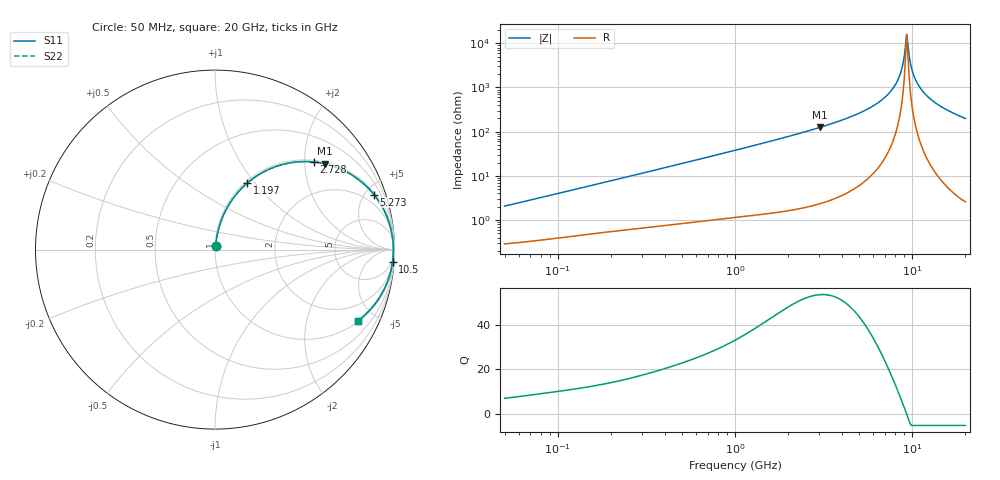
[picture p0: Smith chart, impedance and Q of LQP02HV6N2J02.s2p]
!Murata Part Number: LQP02HV6N2J02
!These Parameters are Measured in Series Mode Connection
!  o--[Z]--o
!Port1  Port2
!  o-------o
!Freq. Start=50[MHz] Stop=20[GHz], 401[Steps]
# Hz S RI R 50
!Freq.(Hz) S11(Real) S11(Imag) S21(Real) S21(Imag) S12(Real) S12(Imag) S22(Real) S22(Imag)
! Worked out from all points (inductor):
!   401 points, 50 MHz to 20 GHz, reference 50 ohm
!   read as one part in series: L = 6.45 nH near 51.52 MHz
!   highest Q = 53.3 at 3.03 GHz (marker M1), where L = 6.6 nH
!   self-resonance near 9.317 GHz
!   S11 on the Smith chart (normalised r, x): 50 MHz: 1.01, +0.04; 1.197 GHz: 1.02, +0.91; 2.728 GHz: 1.04, +2.22; 5.273 GHz: 1.14, +5.74; 10.5 GHz: 4, -29; 20 GHz: 1.05, -3.97
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5e7  0.0033 0.0204  0.9967 -0.0204  0.9967 -0.0204  0.0033 0.0204
1.364002e8  0.0074 0.0531  0.9926 -0.0531  0.9926 -0.0531  0.0074 0.0531
3.721004e8  0.0266 0.1374  0.9734 -0.1374  0.9734 -0.1374  0.0266 0.1374
1e9  0.1329 0.3247  0.8671 -0.3247  0.8671 -0.3247  0.1329 0.3247
1.196911e9  0.178 0.3691  0.822 -0.3691  0.822 -0.3691  0.178 0.3691
2.728004e9  0.5501 0.4881  0.4499 -0.4881  0.4499 -0.4881  0.5501 0.4881
3.029571e9  0.6104 0.4784  0.3896 -0.4784  0.3896 -0.4784  0.6104 0.4784
5.273168e9  0.8859 0.306  0.1141 -0.306  0.1141 -0.306  0.8859 0.306
6.406762e9  0.9464 0.2093  0.0536 -0.2093  0.0536 -0.2093  0.9464 0.2093
7.442007e9  0.9764 0.1282  0.0236 -0.1282  0.0236 -0.1282  0.9764 0.1282
8.020766e9  0.9859 0.0862  0.0141 -0.0862  0.0141 -0.0862  0.9859 0.0862
8.516016e9  0.9908 0.0522  0.00917 -0.0522  0.00917 -0.0522  0.9908 0.0522
8.774992e9  0.9924 0.0352  0.00759 -0.0352  0.00759 -0.0352  0.9924 0.0352
9.178299e9  0.9937 0.00945  0.00634 -0.00945  0.00634 -0.00945  0.9937 0.00945
9.316812e9  0.9938 0.000863  0.00622 -0.000863  0.00622 -0.000863  0.9938 0.000863
9.457416e9  0.9937 -0.00772  0.00625 0.00772  0.00625 0.00772  0.9937 -0.00772
1.004137e10  0.9921 -0.0421  0.00787 0.0421  0.00787 0.0421  0.9921 -0.0421
1.050288e10  0.9893 -0.0678  0.0107 0.0678  0.0107 0.0678  0.9893 -0.0678
1.149051e10  0.9797 -0.1189  0.0203 0.1189  0.0203 0.1189  0.9797 -0.1189
1.314879e10  0.9548 -0.1938  0.0452 0.1938  0.0452 0.1938  0.9548 -0.1938
1.597544e10  0.8967 -0.2957  0.1033 0.2957  0.1033 0.2957  0.8967 -0.2957
2e10  0.7944 -0.3976  0.2056 0.3976  0.2056 0.3976  0.7944 -0.3976
